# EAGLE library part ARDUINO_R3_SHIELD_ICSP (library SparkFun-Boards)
Arduino R3 Shield Footprint with ICSP Header Includes pins for 6-pin (2x3) ICSP Header. Compatible with Leonardo boards that require SPI pin connections via this header. SparkFun Products: CryptoShield microSD Shield
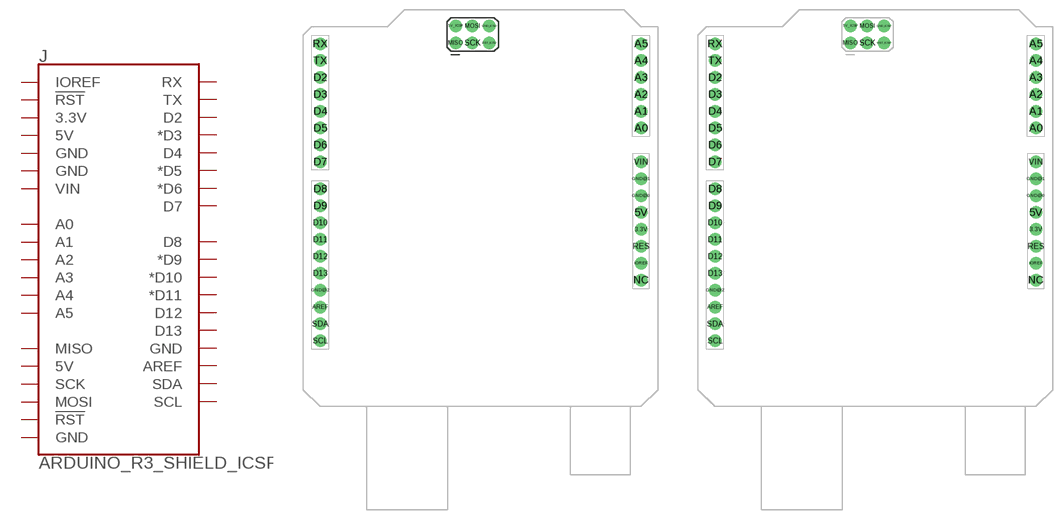
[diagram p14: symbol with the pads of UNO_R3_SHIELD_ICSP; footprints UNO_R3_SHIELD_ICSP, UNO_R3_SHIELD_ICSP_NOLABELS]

Designator prefix J

## ARDUINO_R3_SHIELD_ICSP  [UNO_R3_SHIELD_ICSP]
3.3V  3.3V
5V  5V
5V_ICSP  5V
A0  A0
A1  A1
A2  A2
A3  A3
A4  A4
A5  A5
AREF  AREF
D2  D2
D3  *D3
D4  D4
D5  *D5
D6  *D6
D7  D7
D8  D8
D9  *D9
D10  *D10
D11  *D11
D12  D12
D13  D13
GND@0  GND
GND@1  GND
GND@2  GND
GND_ICSP  GND
IOREF  IOREF
MISO  MISO
MOSI  MOSI
RES  !RST!
RST_ICSP  !RST!
RX  RX
SCK  SCK
SCL  SCL
SDA  SDA
TX  TX
VIN  VIN

## ARDUINO_R3_SHIELD_ICSP-NO_LABELS  [UNO_R3_SHIELD_ICSP_NOLABELS]
Pads as for UNO_R3_SHIELD_ICSP

## Footprint UNO_R3_SHIELD_ICSP (pad centres in mm)
drill 1.016 pad 1.88: 3.3V 50.8,26.67; 5V 50.8,29.21; 5V_ICSP 22.91,57.29; A0 50.8,41.91; A1 50.8,44.45; A2 50.8,46.99; A3 50.8,49.53; A4 50.8,52.07; A5 50.8,54.61; AREF 2.54,14.986; D2 2.54,49.53; D3 2.54,46.99; D4 2.54,44.45; D5 2.54,41.91; D6 2.54,39.37; D7 2.54,36.83; D8 2.54,32.766; D9 2.54,30.226; D10 2.54,27.686; D11 2.54,25.146; D12 2.54,22.606; D13 2.54,20.066; GND@0 50.8,31.75; GND@1 50.8,34.29; GND@2 2.54,17.526; GND_ICSP 27.99,57.29; IOREF 50.8,21.59; MISO 22.91,54.75; MOSI 25.45,57.29; NC 50.8,19.05; RES 50.8,24.13; RST_ICSP 27.99,54.75; RX 2.54,54.61; SCK 25.45,54.75; SCL 2.54,9.906; SDA 2.54,12.446; TX 2.54,52.07; VIN 50.8,36.83

## Footprint UNO_R3_SHIELD_ICSP_NOLABELS (pad centres in mm)
drill 1.016 pad 1.88: 3.3V 50.8,26.67; 5V 50.8,29.21; 5V_ICSP 22.91,57.29; A0 50.8,41.91; A1 50.8,44.45; A2 50.8,46.99; A3 50.8,49.53; A4 50.8,52.07; A5 50.8,54.61; AREF 2.54,14.986; D2 2.54,49.53; D3 2.54,46.99; D4 2.54,44.45; D5 2.54,41.91; D6 2.54,39.37; D7 2.54,36.83; D8 2.54,32.766; D9 2.54,30.226; D10 2.54,27.686; D11 2.54,25.146; D12 2.54,22.606; D13 2.54,20.066; GND@0 50.8,31.75; GND@1 50.8,34.29; GND@2 2.54,17.526; GND_ICSP 27.99,57.29; IOREF 50.8,21.59; MISO 22.91,54.75; MOSI 25.45,57.29; NC 50.8,19.05; RES 50.8,24.13; RST_ICSP 27.99,54.75; RX 2.54,54.61; SCK 25.45,54.75; SCL 2.54,9.906; SDA 2.54,12.446; TX 2.54,52.07; VIN 50.8,36.83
